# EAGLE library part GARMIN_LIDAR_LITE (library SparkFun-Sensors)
This is a device for the Garmin LIDAR Lite v4.
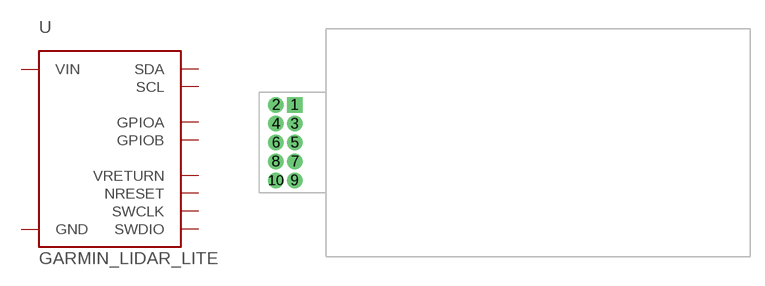
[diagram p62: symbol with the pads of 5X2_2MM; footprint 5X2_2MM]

Designator prefix U

## GARMIN_LIDAR_LITE5X2_2MM (PROD_ID: SEN-14784, CONN-15822)  [5X2_2MM]
1  VIN  pwr
2  GND  pwr
3  SDA
4  SCL
5  GPIOA  out
6  GPIOB  out
7  VRETURN
8  NRESET
9  SWCLK
10  SWDIO

## Footprint 5X2_2MM (pad centres in mm)
drill 1.016 pad 1.651 square: 1 1,4
drill 1.016 pad 1.651: 2 -1,4; 3 1,2; 4 -1,2; 5 1,0; 6 -1,0; 7 1,-2; 8 -1,-2; 9 1,-4; 10 -1,-4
